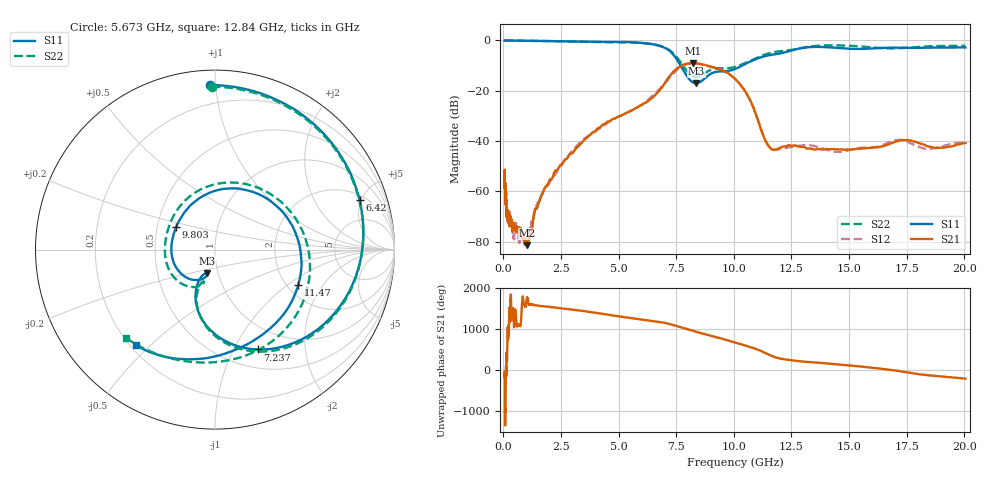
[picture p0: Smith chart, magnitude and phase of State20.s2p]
# Hz S DB R 50
!freq MagS11 AngS11 MagS21 AngS21 MagS12 AngS12 MagS22 AngS22
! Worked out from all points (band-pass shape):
!   1601 points, 50 MHz to 20.05 GHz, reference 50 ohm
!   highest |S21| = -9.05 dB at 8.22 GHz (marker M1); lowest = -81.5 dB at 1.036 GHz (marker M2)
!   |S21| within 3 dB of the highest: 7.419 GHz to 9.553 GHz (2.133 GHz wide, 25.1 % of centre)
!   lowest |S11| = -17.0 dB at 8.376 GHz (marker M3), VSWR 1.33, Z = 44.1 - j12 ohm
!   |S11| at or under -10 dB: 7.69 GHz to 10.36 GHz (2.666 GHz wide, 29.5 % of centre)
!   |S22| runs from -14.5 to 0.0 dB; largest |S21 - S12| = 0.022
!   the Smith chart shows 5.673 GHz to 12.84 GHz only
!   S11 on the Smith chart (normalised r, x): 5.673 GHz: 0.08, +0.97; 6.42 GHz: 2.40, +4.84; 7.237 GHz: 0.71, -1.25; 9.803 GHz: 0.63, +0.17; 11.47 GHz: 2.30, -1.20; 12.84 GHz: 0.22, -0.45
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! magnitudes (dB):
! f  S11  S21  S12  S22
! 50 MHz  0.0  -55.8  -52.0  0.0
! 71.91 MHz  0.0  -57.8  -57.6  0.0
! 78.67 MHz  0.0  -65.2  -60.0  0.0
! 112.3 MHz  0.0  -60.7  -64.4  0.0
! 135.9 MHz  0.0  -67.3  -65.5  0.0
! 369.6 MHz  0.0  -73.4  -73.5  0.0
! 449.1 MHz  0.0  -73.6  -78.2  0.0
! 535.6 MHz  -0.1  -75.6  -73.0  -0.1
! 1.005 GHz  -0.1  -79.9  -80.4  -0.1
! 1.036 GHz  -0.1  -81.5  -80.3  -0.1
! 2.722 GHz  -0.3  -47.1  -47.0  -0.4
! 5.673 GHz  -0.7  -27.2  -27.3  -0.8
! 6.42 GHz  -1.4  -23.1  -22.4  -1.4
! 7.237 GHz  -4.4  -13.9  -14.6  -4.1
! 7.402 GHz  -5.9  -12.2  -12.9  -5.4
! 8.22 GHz  -16.6  -9.0  -9.1  -14.2
! 8.376 GHz  -17.0  -9.2  -9.1  -14.5
! 9.803 GHz  -12.0  -13.4  -13.5  -11.0
! 10.57 GHz  -9.0  -21.4  -21.3  -8.7
! 11.47 GHz  -5.9  -41.5  -41.4  -5.2
! 12.84 GHz  -3.2  -42.2  -41.8  -3.1
! 20.05 GHz  -2.8  -40.8  -40.5  -2.1
